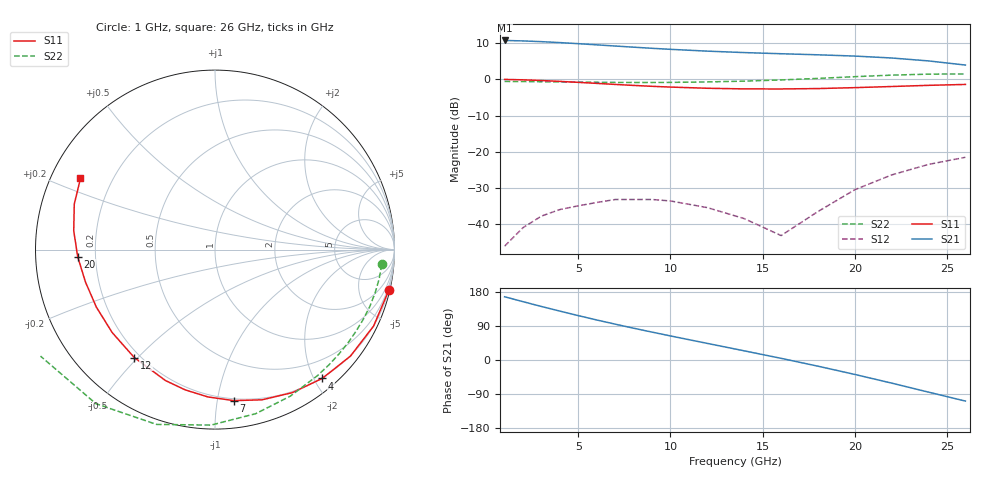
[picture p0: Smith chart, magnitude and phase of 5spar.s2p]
!  MwT-5  S-PARAMETERS
! FREQ  VDS = 6.0 VOLTS,  IDS = 0.6 IDSS = 35 MA
!  S11  S21  S12  S22
#GHZ S MA R 50
!  MAG  ANG  MAG  ANG  MAG  ANG  MAG  ANG
!UPDATED  6/6/97
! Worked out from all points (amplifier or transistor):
!   18 points, 1 GHz to 26 GHz, reference 50 ohm
!   highest |S21| = 10.7 dB at 1 GHz (marker M1)
!   |S21| within 3 dB of that: start of sweep to 12.28 GHz
!   unconditionally stable (mu >= 1): 10.63 GHz to 14.34 GHz
!   at 4 GHz: K = 0.42, MSG = 23.0 dB, |S12| = -35.9 dB
!   at 10 GHz: K = 0.97, MSG = 20.9 dB, |S12| = -33.6 dB
!   at 26 GHz: K = -1.36, MSG = 12.7 dB, |S12| = -21.5 dB
!   S11 on the Smith chart (normalised r, x): 1 GHz: 0.20, -8.77; 4 GHz: 0.19, -2.12; 7 GHz: 0.19, -1.11; 12 GHz: 0.18, -0.49; 20 GHz: 0.13, -0.03; 26 GHz: 0.09, +0.25
1  0.995 -13.0  3.425 166.9  0.005 81.4  0.933 -5.1
2  0.981 -25.7  3.375 153.9  0.009 72.9  0.929 -10.2
3  0.96 -38.2  3.297 141.2  0.013 64.7  0.924 -15.2
4  0.934 -50.2  3.2 129.0  0.016 57.0  0.919 -20.2
5  0.906 -61.6  3.092 117.1  0.018 49.7  0.913 -25.1
6  0.877 -72.6  2.98 105.6  0.02 42.9  0.908 -30.0
7  0.848 -82.9  2.87 94.6  0.022 36.6  0.905 -35.0
8  0.822 -92.7  2.766 83.9  0.022 30.9  0.903 -40.2
9  0.799 -102.0  2.67 73.6  0.022 25.6  0.903 -45.4
10  0.78 -110.7  2.584 63.5  0.021 21.0  0.905 -50.9
12  0.751 -126.8  2.44 43.8  0.017 14.3  0.918 -62.8
14  0.736 -141.2  2.331 24.2  0.012 16.1  0.942 -76.1
16  0.7347 -154.2  2.247 4.4  0.007 58.9  0.978 -91.3
18  0.744 -166.0  2.172 -16.3  0.015 107.2  1.027 -108.5
20  0.766 -177.0  2.086 -38.1  0.03 108.4  1.085 -127.7
22  0.794 172.4  1.963 -61.0  0.048 98.7  1.139 -148.6
24  0.824 162.1  1.789 -84.8  0.067 85.5  1.176 -170.2
26  0.848 152.1  1.569 -108.4  0.084 71.4  1.183 168.8
